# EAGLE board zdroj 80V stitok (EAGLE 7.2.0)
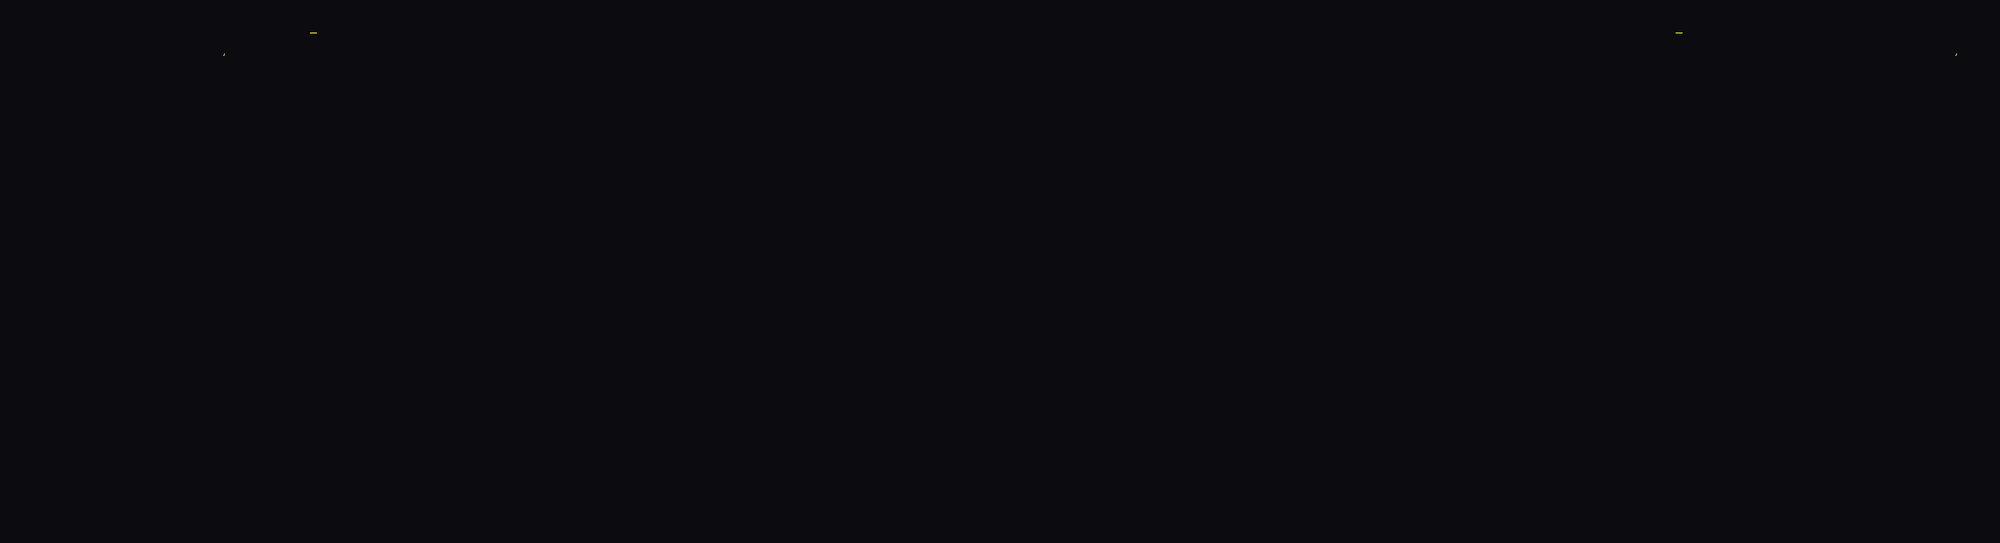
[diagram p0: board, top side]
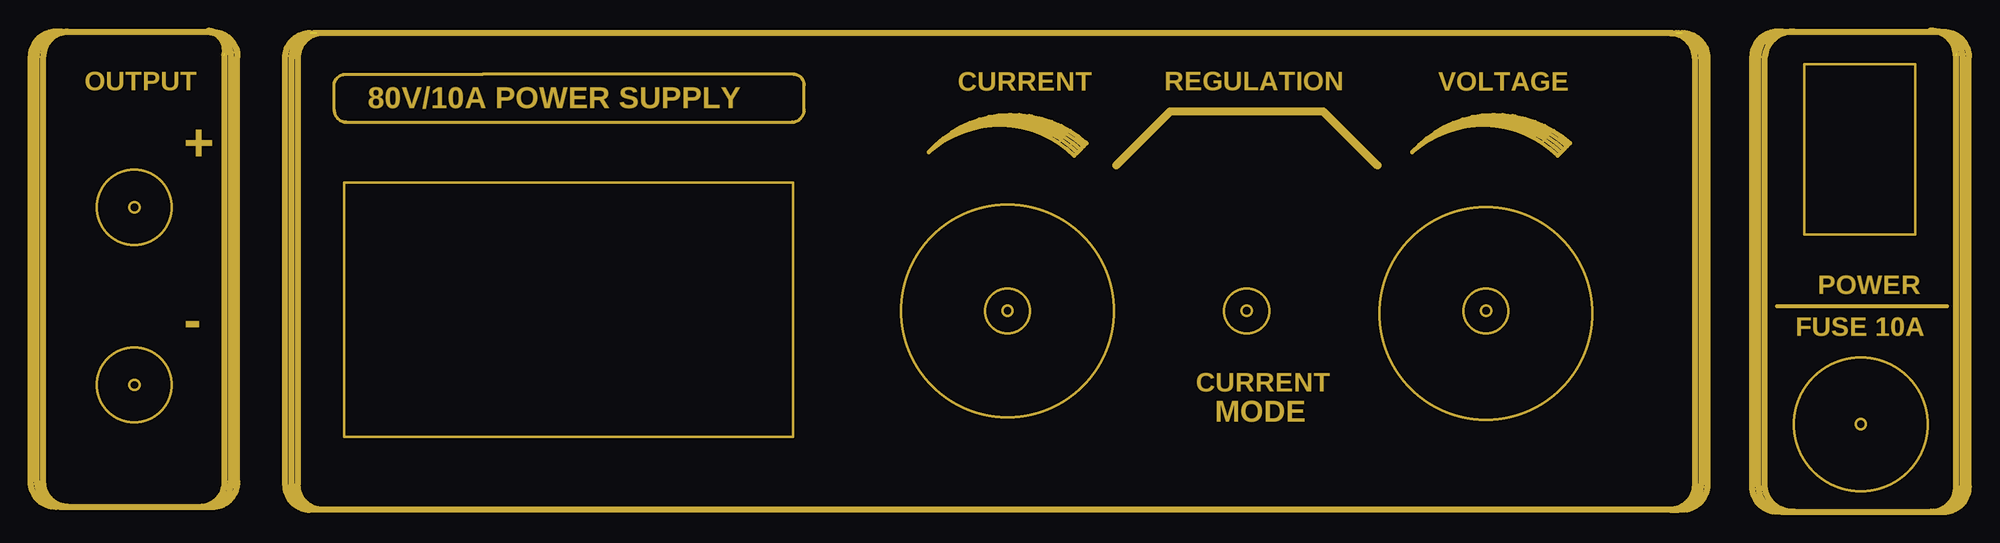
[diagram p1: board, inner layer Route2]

No outline drawn. Coordinates in mm, seen from the top.
Copper layers (1*16): Top 0.035mm / dielectric 1.5mm / Bottom 0.035mm
Design rules "default": minimum track width 10mil, minimum drill 24mil, track to track 8mil, track to pad 8mil, pad to pad 8mil, via to via 8mil, smd to smd 8mil, copper to edge 40mil, drill to drill 8mil, minimum pad ring 10mil, minimum via ring 8mil, stop-mask expansion 4mil, vias tented up to drill 0mil, thermal gap 10mil

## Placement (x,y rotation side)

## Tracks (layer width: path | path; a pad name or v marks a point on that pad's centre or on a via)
N$1
  Route2 0.406: 39.04,-47.24 38.72,-47.55 | 38.4,-47.87 38.72,-47.55 | 38.08,-48.19 38.4,-47.87 | 39.04,-47.24 38.72,-47.08 arc90 23.02,-48.17 | 38.08,-48.19 37.77,-48.51 arc87 23.02,-48.17 | 23.02,-48.17 arc-90 39.04,-47.24 | 23.02,-48.17 arc-90 39.04,-47.24 | 23.02,-48.17 arc-87 38.08,-48.19 | 23.02,-48.17 arc-87 38.08,-48.19 | 23.02,-48.17 arc-87 38.4,-47.87 | 23.02,-48.17 arc-87 38.72,-47.55 | 23.02,-48.17 arc-87 39.04,-47.24 | 23.02,-48.17 arc-87 39.04,-47.24
N$2
  Route2 0.61: -47.05,-38.48 arc90 -49.59,-35.95 -50.23,-35.95 arc-90 -47.69,-38.48
N$3
  Route2 0.406: 88.04,-47.24 87.72,-47.55 | 87.4,-47.87 87.72,-47.55 | 87.08,-48.19 87.4,-47.87 | 88.04,-47.24 87.72,-47.08 arc90 72.02,-48.17 | 87.08,-48.19 86.77,-48.51 arc87 72.02,-48.17 | 72.02,-48.17 arc-90 88.04,-47.24 | 72.02,-48.17 arc-90 88.04,-47.24 | 72.02,-48.17 arc-87 87.08,-48.19 | 72.02,-48.17 arc-87 87.08,-48.19 | 72.02,-48.17 arc-87 87.4,-47.87 | 72.02,-48.17 arc-87 87.72,-47.55 | 72.02,-48.17 arc-87 88.04,-47.24 | 72.02,-48.17 arc-87 88.04,-47.24
N$4  (1 unrouted)
  Route2 0.61: -47.05,-38.48 -47.05,-81.58 arc-90 -49.59,-84.12 -50.23,-84.12 | -47.69,-38.17 -47.69,-81.58 arc-90 -50.23,-84.12 | -48.33,-38.17 -48.33,-81.58 arc-90 -50.87,-84.12 | -64.2,-35.95 arc90 -66.74,-38.48 -66.74,-81.58 arc90 -64.2,-84.12 | -64.2,-35.95 -50.5,-35.95 | -50.87,-84.12 -50.23,-84.12 | -64.2,-84.12 -50.87,-84.12 | -64.83,-35.95 -65.47,-35.95 arc90 -68.01,-38.48 -68.01,-81.58 arc90 -65.47,-84.12 -64.83,-84.12 | -64.83,-35.95 -64.2,-35.95 | -64.83,-35.95 arc90 -67.38,-38.48 -67.38,-81.58 arc90 -64.83,-84.12 | -64.83,-84.12 -64.2,-84.12 | -48.38,-38.37 arc90 -49.91,-35.83
N$5
  Route2 0.61: -50.5,-35.95 -49.59,-35.95
N$6
  Route2 0.813: 68.5,-49.5 63,-44 47.5,-44 42,-49.5
N$7
  Route2 0.254: 111.75,-56.5 111.75,-39.25 123,-39.25 123,-56.5 111.75,-56.5
N$8
  Route2 0.406: 109,-63.75 126.25,-63.75
N$9
  Route2 0.254: -36.25,-77 -36.25,-51.25 9.25,-51.25 9.25,-77 -36.25,-77
N$39  (1 unrouted)
  Route2 0.61: 128.44,-38.48 128.44,-82.08 arc-90 125.91,-84.62 125.27,-84.62 | 127.81,-38.17 127.81,-82.08 arc-90 125.27,-84.62 | 127.17,-38.17 127.17,-82.08 arc-90 124.64,-84.62 | 110.8,-35.95 arc90 107.76,-38.48 107.76,-82.08 arc90 110.8,-84.62 | 110.8,-35.95 124,-35.95 | 124.64,-84.62 125.27,-84.62 | 110.8,-84.62 124.64,-84.62 | 109.67,-35.95 109.03,-35.95 arc90 106.49,-38.48 106.49,-82.08 arc90 109.03,-84.62 109.67,-84.62 | 109.67,-35.95 110.8,-35.95 | 109.67,-35.95 arc90 107.12,-38.48 107.12,-82.08 arc90 109.67,-84.62 | 109.67,-84.62 110.8,-84.62 | 127.12,-38.37 arc90 124.58,-35.83
N$42  (2 unrouted)
  Route2 0.61: 98.14,-36.07 98.77,-36.07 arc-90 101.31,-38.61 101.31,-81.88 arc-90 98.77,-84.42 98.14,-84.42 | 98.14,-36.07 -38.41,-36.07 | -38.41,-36.07 -39.05,-36.07 arc90 -41.59,-38.61 -41.59,-81.88 arc90 -39.05,-84.42 -38.41,-84.42 | 98.14,-84.42 -38.41,-84.42 | -39.68,-84.42 arc-90 -42.22,-81.88 -42.22,-38.61 arc-90 -39.68,-36.07 | 98.14,-36.07 arc-90 100.67,-38.61 100.67,-81.88 arc-90 98.14,-84.42 | -38.41,-84.42 arc-90 -40.95,-81.88 -40.95,-38.61 arc-90 -38.41,-36.07 | 99.41,-84.42 arc90 101.94,-81.88 101.94,-38.61 arc90 99.41,-36.07
N$136
  Route2 0.61: 124,-35.95 125.91,-35.95
N$137
  Route2 0.61: 125.27,-35.95 125.91,-35.95 arc-90 128.44,-38.48 | 125.27,-35.95 124.32,-35.95 | 127.81,-38.48 arc90 125.27,-35.95
N$163
  Route2 0.305: -22.19,-40.25 9.29,-40.25 arc-90 10.4,-41.36 10.4,-43.83 arc-90 9.13,-45.1 -36,-45.1 arc-90 -37.27,-43.83 -37.27,-41.36 arc-90 -36,-40.25 -22.19,-40.25
(copper drawn outside any net)
  shapes: Route2 circle x14

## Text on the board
Route2: OUTPUT | CURRENT | REGULATION | VOLTAGE | 80V/10A POWER SUPPLY | + | POWER | - | FUSE 10A | CURRENT | MODE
